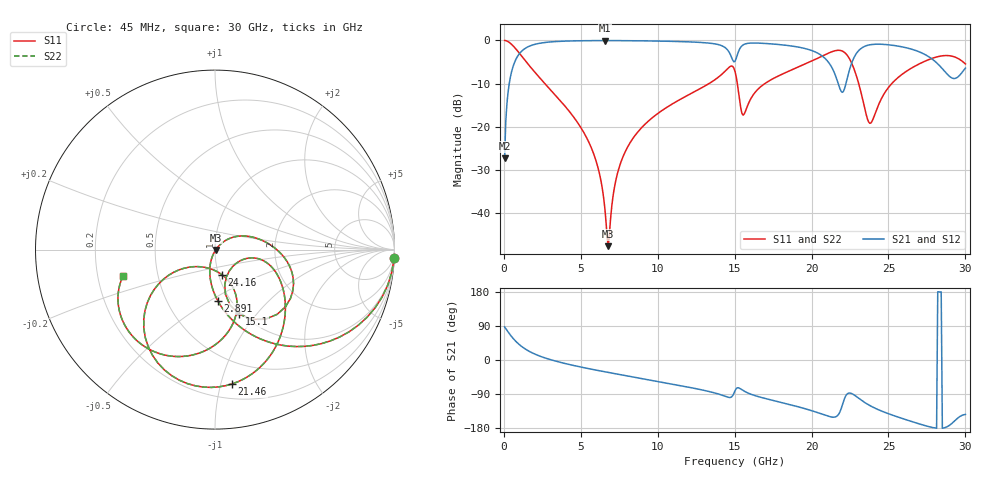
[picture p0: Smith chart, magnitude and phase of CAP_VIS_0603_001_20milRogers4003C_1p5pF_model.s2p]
! S-parameter model data by Modelithics Inc.  support@modelithics.com  813-866-6335  Tampa FL USA
! S-Parameter data specifications:
! Substrate: 20-mil Rogers 4003C, substrate thickness, H=0.508mm, Dielectric constant, Er=3.75
! PCB Mounting Pad Footprint: Pad width, PadW=0.90mm , Pad length, PadL=1.00mm , Pad gap, PadG (edge-to-edge)=1.00mm , Reference planes=3.0mm apart
! Created Wed Nov 18 13:18:29 2015
# hz S ma R 50
! 2 Port Network Data from SP1.SP block
! freq  magS11  angS11  magS21  angS21  magS12  angS12  magS22  angS22
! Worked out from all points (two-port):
!   401 points, 45 MHz to 30 GHz, reference 50 ohm
!   highest |S21| = -0.04 dB at 6.56 GHz (marker M1); lowest = -27.3 dB at 45 MHz (marker M2)
!   |S21| within 3 dB of the highest: 1.014 GHz to 14.69 GHz (13.67 GHz wide, 174 % of centre); 15.2 GHz to 20.45 GHz (5.243 GHz wide, 29.4 % of centre)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
!   lowest |S11| = -47.6 dB at 6.785 GHz (marker M3), VSWR 1.01, Z = 50.4 - j0.194 ohm
!   |S11| at or under -10 dB: 2.664 GHz to 13.33 GHz (10.67 GHz wide, 133 % of centre); 15.17 GHz to 16.96 GHz (1.786 GHz wide, 11.1 % of centre); 23.06 GHz to 25.21 GHz (2.15 GHz wide, 8.91 % of centre)
!   |S22| runs from -47.6 to 0.0 dB; largest |S21 - S12| = 0
!   S11 on the Smith chart (normalised r, x): 45 MHz: 1, -43; 2.891 GHz: 0.87, -0.54; 15.1 GHz: 0.97, -0.82; 21.46 GHz: 0.31, -1.08; 24.16 GHz: 1.04, -0.30; 30 GHz: 0.31, -0.13
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4.5e7  0.9991 -2.7  0.04321 87.3  0.04321 87.3  0.9991 -2.7
3.4455e8  0.949 -20.0  0.315 70.0  0.315 70.0  0.949 -20.0
7.189875e8  0.8195 -38.4  0.5722 51.6  0.5722 51.6  0.8195 -38.4
2.890725e9  0.2854 -86.9  0.9557 2.6  0.9557 2.6  0.2854 -86.9
5.062462e9  0.09399 -107.0  0.9917 -19.1  0.9917 -19.1  0.09399 -107.0
6.560212e9  0.0114 -100.3  0.9953 -31.1  0.9953 -31.1  0.0114 -100.3
6.784875e9  0.004146 -27.7  0.9953 -32.8  0.9953 -32.8  0.004146 -27.7
7.758412e9  0.0458 44.2  0.9937 -40.1  0.9937 -40.1  0.0458 44.2
1.007992e10  0.1458 30.6  0.9826 -57.1  0.9826 -57.1  0.1458 30.6
1.359964e10  0.3392 0.7  0.9188 -85.8  0.9188 -85.8  0.3392 0.7
1.50225e10  0.4388 -62.3  0.5734 -81.3  0.5734 -81.3  0.4388 -62.3
1.509739e10  0.3827 -69.7  0.6172 -75.8  0.6172 -75.8  0.3827 -69.7
1.56216e10  0.1404 -33.2  0.9007 -82.2  0.9007 -82.2  0.1404 -33.2
2.003996e10  0.5803 -49.5  0.7602 -134.2  0.7602 -134.2  0.5803 -49.5
2.146282e10  0.7544 -82.8  0.4298 -150.9  0.4298 -150.9  0.7544 -82.8
2.198704e10  0.7541 -105.3  0.2506 -120.8  0.2506 -120.8  0.7541 -105.3
2.251125e10  0.5919 -132.1  0.4862 -87.3  0.4862 -87.3  0.5919 -132.1
2.370945e10  0.1137 -119.4  0.8839 -118.4  0.8839 -118.4  0.1137 -119.4
2.415878e10  0.1465 -74.1  0.9037 -127.8  0.9037 -127.8  0.1465 -74.1
2.505742e10  0.2938 -66.0  0.8878 -142.6  0.8878 -142.6  0.2938 -66.0
2.805292e10  0.6376 -111.1  0.5665 -179.5  0.5665 -179.5  0.6376 -111.1
3e10  0.5342 -163.9  0.4782 -143.6  0.4782 -143.6  0.5342 -163.9
